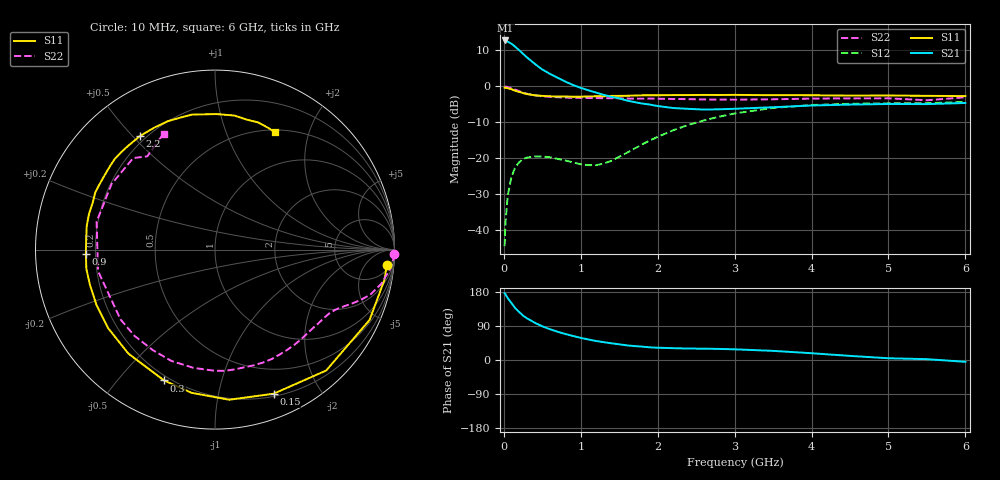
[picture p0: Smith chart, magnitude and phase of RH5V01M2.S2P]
! SIEMENS Small Signal Semiconductors
! BFR106
! Si NPN RF Bipolar Junction Transistor in SOT23
! VCE = 5 V  IC = 1.2 mA
! Common Emitter S-Parameters:  August  1996
# GHz  S  MA  R  50
!  f  S11  S21  S12  S22
! GHz  MAG  ANG  MAG  ANG  MAG  ANG  MAG  ANG
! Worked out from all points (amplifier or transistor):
!   36 points, 10 MHz to 6 GHz, reference 50 ohm
!   highest |S21| = 12.8 dB at 20 MHz (marker M1)
!   |S21| within 3 dB of that: start of sweep to 213.7 MHz
!   unconditionally stable (mu >= 1): 849.5 MHz to 1.868 GHz; 3.256 GHz to end of sweep
!   at 250 MHz: K = 0.27, MSG = 14.6 dB, |S12| = -20.2 dB
!   at 1.4 GHz: K = 1.35, MAG = 5.4 dB, |S12| = -20.7 dB
!   at 6 GHz: K = 1.02, MAG = -1.0 dB, |S12| = -4.3 dB
!   S11 on the Smith chart (normalised r, x): 10 MHz: 9, -19; 150 MHz: 0.23, -1.46; 300 MHz: 0.18, -0.67; 900 MHz: 0.16, -0.02; 2.2 GHz: 0.18, +0.53; 6 GHz: 0.53, +1.50
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0.01  0.9612 -5.0  4.342 176.2  0.006 88.7  0.9999 -1.4
0.02  0.9594 -10.0  4.362 173.7  0.012 85.4  0.9979 -2.6
0.05  0.9461 -24.5  4.204 163.6  0.0302 75.6  0.9812 -6.4
0.1  0.9152 -47.4  3.918 150.0  0.0561 64.1  0.9444 -11.8
0.15  0.8668 -67.9  3.556 136.3  0.0754 53.2  0.9007 -16.2
0.2  0.8402 -84.6  3.187 126.5  0.0884 45.1  0.8595 -19.0
0.25  0.8086 -99.3  2.841 117.1  0.0977 38.2  0.8217 -21.4
0.3  0.7822 -111.3  2.54 110.1  0.1025 33.7  0.7929 -23.2
0.4  0.7541 -129.8  2.071 98.6  0.1065 26.4  0.753 -26.2
0.5  0.7389 -143.7  1.721 88.9  0.106 22.0  0.7301 -29.0
0.7  0.7238 -164.2  1.318 74.4  0.0982 19.5  0.7075 -35.5
0.9  0.7198 -178.2  1.047 63.3  0.0876 24.1  0.6944 -42.3
1.1  0.7269 169.4  0.883 54.2  0.0803 36.0  0.6906 -50.1
1.3  0.7295 159.2  0.763 47.0  0.0847 53.1  0.6865 -58.3
1.6  0.7417 145.8  0.636 38.6  0.1197 71.6  0.6801 -71.3
2.2  0.7585 123.4  0.501 31.2  0.2453 73.7  0.6697 -100.3
2.8  0.7603 104.7  0.481 29.2  0.3798 60.2  0.6574 -133.1
3.5  0.7552 89.5  0.514 24.1  0.5029 41.7  0.6625 -169.6
4.5  0.7453 76.2  0.559 10.8  0.5737 18.4  0.6824 147.6
5  0.7483 71.2  0.57 4.6  0.583 9.8  0.6839 131.8
5.5  0.74 66.2  0.568 2.2  0.5843 5.7  0.6422 126.0
6  0.734 62.9  0.589 -4.8  0.6092 -2.4  0.707 113.9
